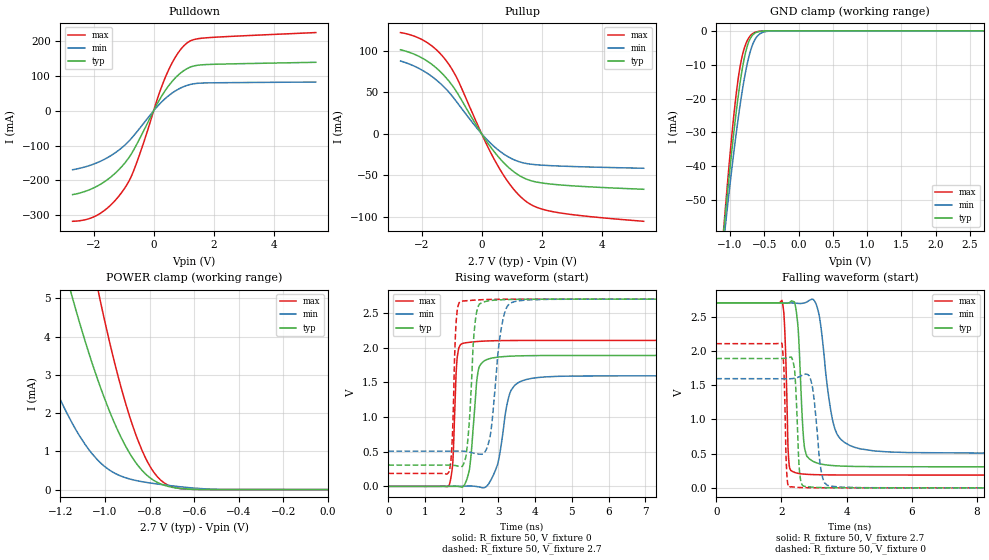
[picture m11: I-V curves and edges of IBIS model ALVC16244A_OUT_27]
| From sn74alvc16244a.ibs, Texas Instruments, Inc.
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[Model]   ALVC16244A_OUT_27
Model_type  3-state
Enable   Active-Low
Vref =   0
Rref =   500
Cref =   50p
Vmeas =   1.5
| variable   typ   min   max
C_comp   2.45pF   2.20pF   2.56pF
| C_pullup   3.51pF   3.04pF   4.30pF
| C_pulldown   4.68pF   2.99pF   6.80pF
| C_tri-state   2.45pF   2.20pF   2.56pF
[Temperature Range]   40   100   -40
| Ambient temperature   25   85   -40
[Voltage range]   2.7   2.7   2.7
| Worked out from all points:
|   slope of the pulldown table from 0 to 0.405 V, typ, clamps not added: 6.69 ohm
|   slope of the pullup table from 0 to 0.405 V, typ, clamps not added: 19.3 ohm
|   GND clamp passes 1 mA (typ) near -0.66 V on its own axis
|   POWER clamp passes 1 mA (typ) near -0.89 V on its own axis
|   rising waveform, R_fixture 50, V_fixture 0: 20-80 % time 167ps typ, 296ps min, 88.5ps max; typ from 0 V to 1.89 V
|   falling waveform, R_fixture 50, V_fixture 2.7: 20-80 % time 143ps typ, 356ps min, 84ps max; typ from 2.7 V to 0.308 V
|   rising waveform, R_fixture 50, V_fixture 2.7: 20-80 % time 154ps typ, 244ps min, 87.6ps max; typ from 0.308 V to 2.7 V
|   falling waveform, R_fixture 50, V_fixture 0: 20-80 % time 101ps typ, 190ps min, 64.8ps max; typ from 1.89 V to 0 V
[GND Clamp]
| ALVC16244A_OUT_27
|   Voltage   I(typ)   I(min)   I(max)
-2.7V     -477.6mA   -435.4mA   -535.6mA
-1.09V    -58.9mA    -61.92mA   -57.94mA
-1.07V    -54.69mA   -58.15mA   -53.03mA
-1.05V    -50.54mA   -54.44mA   -48.21mA
-950mV    -31.09mA   -36.84mA   -26.11mA
-870mV    -17.8mA    -24.35mA   -12.7mA
-825mV    -11.72mA   -18.21mA   -7.72mA
-770mV    -6.129mA   -11.83mA   -3.892mA
-655mV    -955.9uA   -3.345mA   -636.6uA
-560mV    -152.2uA   -821.8uA   -112.4uA
-420mV    -9.47uA    -78.14uA   -9.429uA
2.7V      2.101nA    59.67nA    10.48nA
[POWER Clamp]
| ALVC16244A_OUT_27
|   Voltage   I(typ)   I(min)   I(max)
-2.7V     66.72mA    43.69mA    99.53mA
-1.38V    10.81mA    5.024mA    18.06mA
-1.25V    7.371mA    3.002mA    12.59mA
-1.145V   4.99mA     1.712mA    8.736mA
-1.035V   2.911mA    784.6uA    5.316mA
-1.02V    2.664mA    697.5uA    4.902mA
-940mV    1.512mA    381.5uA    2.931mA
-865mV    729.7uA    243.1uA    1.487mA
-810mV    365.2uA    184.1uA    731.5uA
-750mV    147.6uA    134.7uA    246.1uA
-605mV    6.25uA     41.94uA    4.965uA
-35.59fV  2.101nA    59.67nA    10.48nA
[Pulldown]
| ALVC16244A_OUT_27
|   Voltage   I(typ)   I(min)   I(max)
-2.7V     -241mA     -169.5mA   -317.8mA
-2.19V    -228.9mA   -159mA     -311.3mA
-1.76V    -210.7mA   -144.7mA   -293.9mA
-1.33V    -183.4mA   -123.7mA   -262.3mA
-930mV    -146.9mA   -96.36mA   -218mA
-565mV    -96.6mA    -61.23mA   -149.3mA
150mV     24.79mA    14.91mA    40.94mA
405mV     60.55mA    36.48mA    99.34mA
755mV     97.31mA    58.66mA    158.4mA
1.105V    120.6mA    72.64mA    194.3mA
1.735V    132.7mA    79.91mA    209.5mA
5.4V      139.3mA    82.52mA    224.7mA
[Pullup]
| ALVC16244A_OUT_27
|   Voltage   I(typ)   I(min)   I(max)
-2.7V     101.3mA    87.69mA    122mA
-1.84V    88.28mA    73.59mA    110.6mA
-1.485V   78.58mA    64.13mA    100.6mA
-1.165V   66.78mA    53.2mA     87.42mA
-795mV    48.39mA    36.71mA    65.2mA
5mV       -285.2uA   -208.7uA   -398.2uA
500mV     -25.34mA   -18.03mA   -36.1mA
990mV     -43.56mA   -29.92mA   -63.47mA
1.455V    -54.23mA   -35.75mA   -80.99mA
1.87V     -58.62mA   -37.61mA   -89.33mA
2.495V    -61.46mA   -38.9mA    -94.92mA
5.4V      -67.09mA   -41.72mA   -105.7mA
[Ramp]
| ALVC16244A_OUT_27
| variable   typ   min   max
dV/dt_r   1.14/1.78E-10   0.97/3.08E-10   1.27/9.56E-11
dV/dt_f   1.45/1.47E-10   1.35/3.73E-10   1.53/9.12E-11
R_load = 50
[Rising Waveform]
| ALVC16244A_OUT_27
R_fixture =   50
C_fixture =   0
L_fixture =   0
V_fixture =   0
V_fixture_min = 0
V_fixture_max = 0
|   Time   V(typ)   V(min)   V(max)
0s        277.2pV    442.6pV    174.2pV
1.655ns   796.9uV    -126.8uV   17.8mV
1.755ns   2.822mV    -127.4uV   334.3mV
1.91ns    -1.62mV    311uV      1.972V
2.21ns    243.5mV    6.064mV    2.077V
2.4ns     1.471V     -1.95mV    2.088V
2.97ns    1.862V     305.9mV    2.101V
3.355ns   1.878V     1.393V     2.103V
4.29ns    1.887V     1.579V     2.104V
50ns      1.888V     1.594V     2.105V
[Falling Waveform]
| ALVC16244A_OUT_27
R_fixture =   50
C_fixture =   0
L_fixture =   0
V_fixture =   2.7
V_fixture_min = 2.7
V_fixture_max = 2.7
|   Time   V(typ)   V(min)   V(max)
0s        2.7V       2.7V       2.7V
2.015ns   2.698V     2.7V       2.737V
2.1ns     2.696V     2.7V       2.325V
2.24ns    2.704V     2.7V       325.3mV
2.48ns    2.485V     2.694V     214.7mV
2.63ns    1.099V     2.693V     203.4mV
3.115ns   359.5mV    2.606V     191.7mV
3.7ns     321.4mV    790.1mV    188.3mV
4.86ns    309.6mV    538.4mV    187.1mV
50ns      307.8mV    507.5mV    187mV
[Rising Waveform]
| ALVC16244A_OUT_27
R_fixture =   50
C_fixture =   0
L_fixture =   0
V_fixture =   2.7
V_fixture_min = 2.7
V_fixture_max = 2.7
|   Time   V(typ)   V(min)   V(max)
0s        307.8mV    507.5mV    187mV
1.655ns   307.5mV    508mV      212.8mV
1.74ns    305.4mV    508.3mV    670.8mV
1.855ns   297.4mV    508.6mV    2.425V
2.035ns   304.6mV    507mV      2.674V
2.4ns     2.497V     470.5mV    2.688V
2.83ns    2.682V     953.4mV    2.696V
3.16ns    2.692V     2.486V     2.698V
3.75ns    2.698V     2.687V     2.7V
50ns      2.7V       2.7V       2.7V
[Falling Waveform]
| ALVC16244A_OUT_27
R_fixture =   50
C_fixture =   0
L_fixture =   0
V_fixture =   0
V_fixture_min = 0
V_fixture_max = 0
|   Time   V(typ)   V(min)   V(max)
0s        1.888V     1.594V     2.105V
2.015ns   1.888V     1.592V     2.112V
2.155ns   1.896V     1.592V     294.1mV
2.235ns   1.904V     1.592V     11.24mV
2.405ns   1.72V      1.6V       10.41mV
2.59ns    110.6mV    1.632V     4.962mV
2.95ns    10.27mV    1.474V     1.829mV
3.27ns    3.834mV    139.7mV    829.5uV
3.8ns     1.115mV    11.58mV    241.4uV
50ns      1.457nV    -5.38nV    -673.5pV
